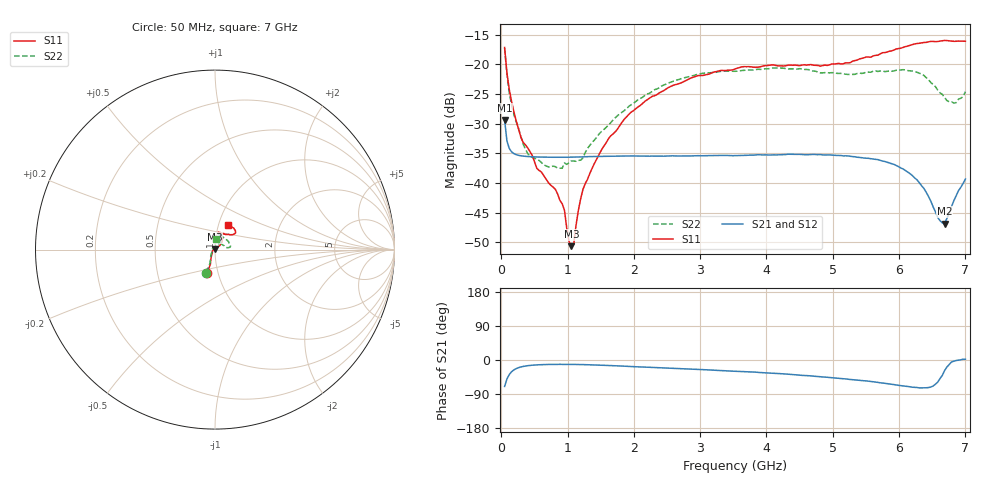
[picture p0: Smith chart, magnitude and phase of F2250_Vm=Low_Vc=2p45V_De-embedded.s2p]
! Integrated Device Technology
! Corporate Headquarters
! 6024 Silver Creek Valley Road
! San Jose, CA 95138  USA
! Phone:  1-408-284-8200
! Toll Free:  1-800-223-1366
! Webpage:  http://www.idt.com/
! Timing and RF Division
! 515 Groton Road, Suite 102
! Westford, MA 01886-6024
! Device:  F2250
! Description: Voltage Variable RF Attenuator
! Frequency:  50.0 -  6000.00 MHz
! Package:  3x3 mm Thin QFN Plastic Package: 16 pin
! Ports:  2 RF, 3 DC
!  Pin  1  = GND
!  Pin  2  = NC
!  Pin  3  = RF1  = Port 1
!  Pin  4  = NC
!  Pin  5  = GND
!  Pin  6  = GND
!  Pin  7  = GND
!  Pin  8  = GND
!  Pin  9  = NC
!  Pin 10  = RF2  = Port 2
!  Pin 11  = NC
!  Pin 12  = GND
!  Pin 13  = GND
!  Pin 14  = VCNTRL
!  Pin 15  = VDD
!  Pin 16  = VMODE
! Vcntrl:  2.450 Volts
! Vmode:  +0.000 Volts
! Vdd:  +3.30  Volts
! Current:  1.176 mA
! Data:  The device was measured on a the F2250 evaluation board which has
!  individual transmission lines to the RF pins.  Data was collected
!  using a calibrated network analyzer.  The evaluation board was
!  de-embedded using a TRL calibration technique.
!  The reference plane is the edge of the package pin.
! Misc:  SN 10
!  Action Tracker AT0258
! Date Measured:  2014-11-26
! Date:  2015-10-15  MJV
! Note:
!  Integrated Device Technology supplies this data as a sample of measured
!  data at the package pin for this product.  Your particular data for this
!  product may vary.
!  Data was taken at 25 degrees C.
!  Integrated Device Technology reserves the right to change this data at anytime.
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# GHz S dB R 50
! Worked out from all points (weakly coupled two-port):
!   201 points, 50 MHz to 7 GHz, reference 50 ohm
!   highest |S21| = -29.41 dB at 50 MHz (marker M1); lowest = -46.9 dB at 6.687 GHz (marker M2)
!   lowest |S11| = -50.7 dB at 1.058 GHz (marker M3), VSWR 1.01, Z = 49.8 + j0.243 ohm
!   |S11| at or under -10 dB: start of sweep to end of sweep
!   |S22| runs from -37.5 to -17.3 dB; largest |S21 - S12| = 6.7e-05
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0.05  -17.18 -108.6  -29.41 -69.8  -29.41 -69.8  -17.27 -111.0
0.08475  -21.44 -107.4  -32.92 -50.4  -32.92 -50.3  -21.75 -110.2
0.15425  -26.23 -116.6  -34.76 -31.1  -34.75 -31.1  -26.81 -122.4
0.29325  -32.21 -127.7  -35.43 -18.5  -35.43 -18.5  -32.10 -137.5
0.3975  -34.09 -141.8  -35.56 -15.0  -35.56 -15.0  -35.03 -160.5
0.5365  -37.56 -155.5  -35.64 -12.8  -35.64 -12.8  -36.05 178.1
0.91875  -43.53 158.1  -35.69 -11.5  -35.68 -11.5  -37.54 133.5
0.9535  -44.65 169.5  -35.68 -11.5  -35.68 -11.5  -36.64 131.1
1.023  -49.92 143.8  -35.68 -11.6  -35.67 -11.6  -36.62 116.0
1.05775  -50.67 123.5  -35.67 -11.6  -35.67 -11.6  -36.29 110.9
1.0925  -50.39 89.6  -35.66 -11.7  -35.66 -11.7  -36.31 106.3
1.162  -44.65 56.9  -35.64 -11.9  -35.64 -11.9  -36.21 95.6
1.2315  -41.12 44.2  -35.61 -12.1  -35.61 -12.1  -35.78 86.0
1.6485  -32.10 42.0  -35.52 -14.6  -35.52 -14.6  -29.88 64.6
2.37825  -24.87 47.3  -35.48 -20.3  -35.48 -20.3  -23.99 56.9
3.525  -20.80 72.5  -35.41 -29.5  -35.40 -29.5  -21.19 74.8
4.7065  -20.16 72.4  -35.20 -42.5  -35.20 -42.5  -21.15 72.3
5.85325  -17.82 40.5  -36.64 -63.2  -36.64 -63.3  -21.13 23.0
6.27025  -16.50 40.1  -39.49 -72.6  -39.51 -72.7  -21.35 9.6
6.68725  -15.99 48.8  -46.85 -27.6  -46.82 -27.3  -25.63 28.4
6.861  -16.13 55.1  -42.18 -1.3  -42.13 -1.2  -26.47 58.0
7  -16.13 63.2  -39.35 1.9  -39.30 1.8  -24.63 83.1
